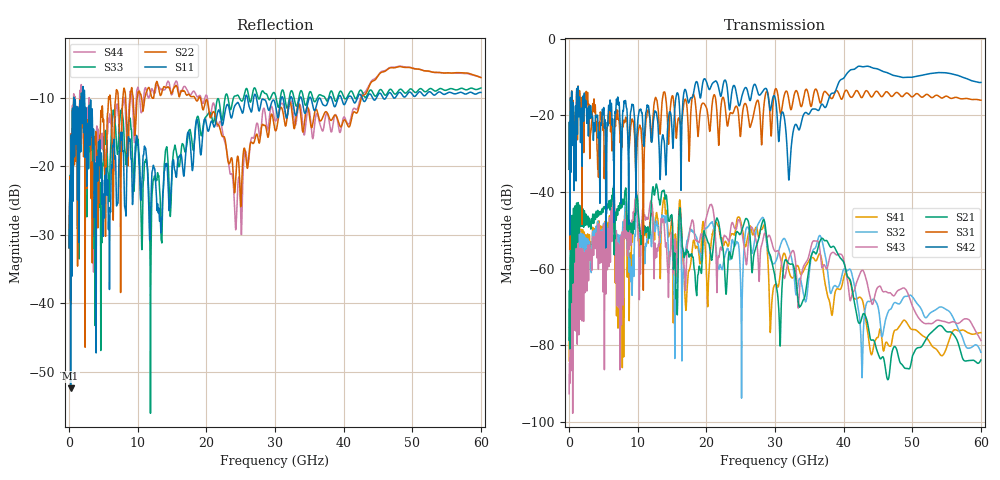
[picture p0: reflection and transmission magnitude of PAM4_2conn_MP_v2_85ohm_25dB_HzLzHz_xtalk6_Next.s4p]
! Info: Touchstone file created by Circ.  Input file=FAB50GbE_2conn_Midplane_Examax_Topo2_v2_85ohm_25dB_HzLzHz.circ
# Hz S RI R 50
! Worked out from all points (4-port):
!   6000 points, 10 MHz to 60 GHz, reference 50 ohm
!   strongest paths, dB at 10 MHz, 15.01 GHz, 30.01 GHz, 45.01 GHz, 60 GHz:
!     S42: -34.0, -24.0, -15.3, -7.9, -11.4
!     S31: -34.1, -15.0, -13.3, -13.9, -16.0
!     S21: -78.7, -46.5, -62.3, -82.2, -83.9
!     S43: -92.7, -51.5, -55.5, -64.8, -78.8
!     S32: -78.5, -52.1, -58.5, -70.0, -81.9
!     S41: -84.1, -46.9, -64.2, -78.0, -76.7
!   lowest |S11| = -52.4 dB at 230 MHz (marker M1), VSWR 1.00, Z = 50.2 - j0.0284 ohm
!   |S11| at or under -10 dB: 2.269 GHz to 25.68 GHz (23.41 GHz wide, 168 % of centre); 27.29 GHz to 30.94 GHz (3.659 GHz wide, 12.6 % of centre); 35.2 GHz to 37.92 GHz (2.713 GHz wide, 7.42 % of centre)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
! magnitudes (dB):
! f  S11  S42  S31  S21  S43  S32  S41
! 10 MHz  -31.9  -34.0  -34.1  -78.7  -92.7  -78.5  -84.1
! 230 MHz  -52.4  -15.9  -15.8  -51.0  -64.1  -57.9  -57.0
! 6.39 GHz  -17.0  -23.4  -28.7  -39.5  -41.1  -39.9  -45.0
! 15.51 GHz  -21.2  -16.1  -22.6  -61.6  -53.2  -64.5  -51.1
! 20.66 GHz  -13.5  -12.5  -21.2  -57.0  -43.2  -48.0  -54.1
! 32.06 GHz  -10.9  -36.5  -16.3  -58.7  -57.2  -55.0  -60.9
! 60 GHz  -9.2  -11.4  -16.0  -83.9  -78.8  -81.9  -76.7
